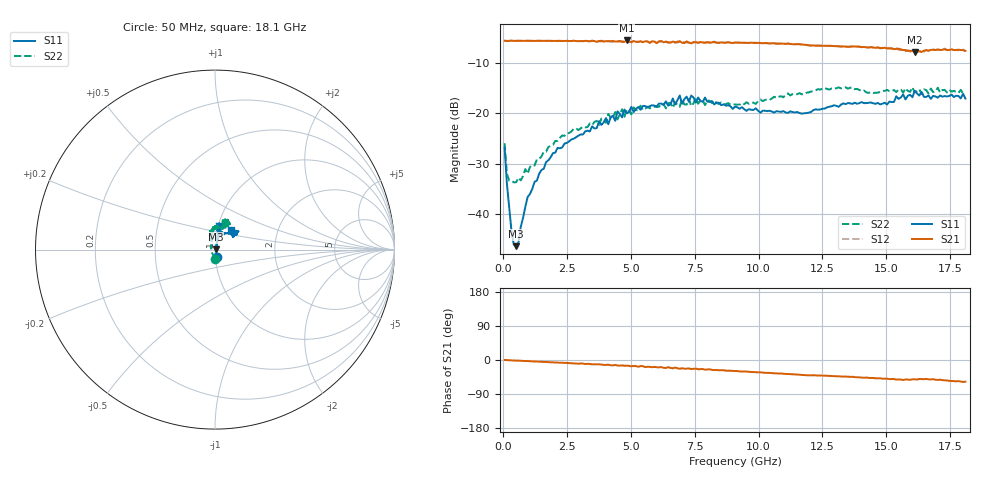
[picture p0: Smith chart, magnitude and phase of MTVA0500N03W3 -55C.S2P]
! Network Analyzer HP8720D.06.14 Serial No. US36140669
!  8 Jul 2005  08:12:55
! Frequency  S11  S21  S12  S22
# HZ  S  DB R 50
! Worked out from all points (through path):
!   201 points, 50 MHz to 18.1 GHz, reference 50 ohm
!   highest |S21| = -5.58 dB at 4.833 GHz (marker M1); lowest = -7.9 dB at 16.11 GHz (marker M2)
!   group delay of S21, straight-line fit = 8.96 ps
!   lowest |S11| = -46.4 dB at 501.2 MHz (marker M3), VSWR 1.01, Z = 50.5 + j0.124 ohm
!   |S11| at or under -10 dB: start of sweep to end of sweep
!   |S22| runs from -33.7 to -14.9 dB; largest |S21 - S12| = 0.021
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5e7  -26.87 -75.3  -5.63 0.2  -5.62 0.2  -25.99 -87.9
1.4025e8  -34.02 -65.2  -5.71 -0.2  -5.67 -0.3  -32.07 -133.1
3.2075e8  -43.46 -41.4  -5.61 -0.8  -5.65 -0.8  -33.43 -168.8
5.0125e8  -46.40 14.8  -5.66 -1.7  -5.66 -1.5  -33.72 170.7
9.525e8  -36.65 62.9  -5.66 -2.8  -5.66 -2.9  -32.02 143.0
1.6745e9  -29.72 69.9  -5.66 -5.2  -5.67 -5.3  -27.64 118.7
3.1185e9  -24.24 78.3  -5.72 -9.5  -5.75 -10.0  -22.68 110.5
4.021e9  -21.00 77.9  -5.72 -13.1  -5.79 -12.2  -21.92 103.4
4.382e9  -21.52 76.1  -5.80 -13.1  -5.75 -14.4  -19.78 103.6
4.47225e9  -19.66 72.5  -5.80 -14.4  -5.72 -13.4  -21.25 106.6
4.83325e9  -20.06 82.0  -5.58 -15.1  -5.73 -16.1  -19.33 94.4
6.09675e9  -18.10 78.1  -5.80 -19.5  -5.71 -19.4  -18.74 94.2
6.7285e9  -18.28 83.1  -5.91 -19.9  -6.10 -20.8  -17.93 88.1
6.909e9  -16.49 81.4  -5.73 -23.1  -5.87 -21.8  -18.74 86.1
6.99925e9  -18.14 80.9  -6.02 -21.9  -6.09 -23.5  -17.26 87.3
7.36025e9  -16.51 75.8  -6.17 -23.9  -5.96 -22.9  -18.61 91.5
7.54075e9  -17.90 76.5  -5.98 -22.6  -5.83 -24.7  -17.03 90.7
9.075e9  -18.74 83.2  -6.01 -29.0  -5.98 -29.0  -18.29 78.8
1.21435e10  -19.41 58.8  -6.58 -40.2  -6.54 -40.3  -15.65 69.4
1.512175e10  -17.72 35.4  -7.18 -50.4  -7.02 -50.0  -15.63 67.6
1.61145e10  -15.58 37.8  -7.88 -51.0  -7.61 -51.1  -15.84 65.7
1.81e10  -17.11 50.6  -7.63 -57.2  -7.81 -57.9  -16.09 70.0
